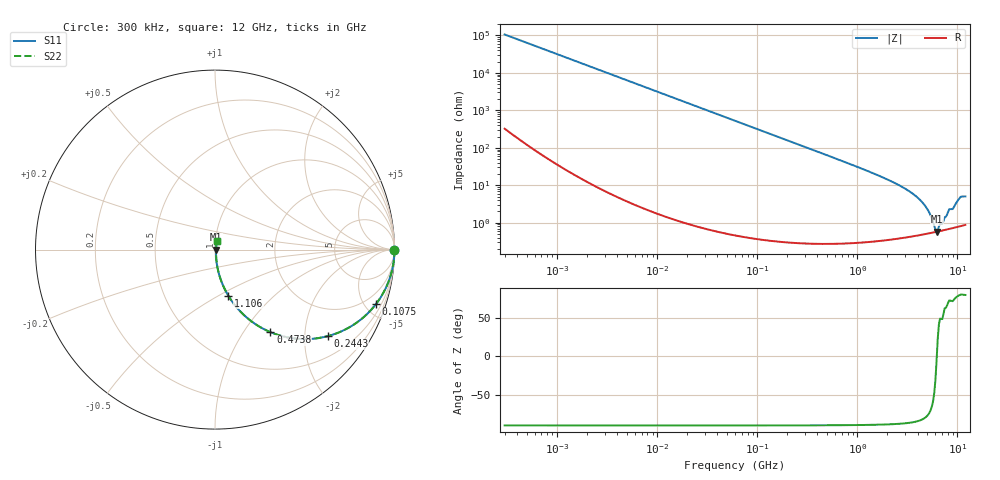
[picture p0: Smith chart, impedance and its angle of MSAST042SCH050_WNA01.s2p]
! MSAST042SCH050_WNA01  S-PARAMETER MODEL  ( General Type )
! Model Generated by TAIYO YUDEN Corporation (http://www.ty-top.com)
! Version 1.0
! TAIYO YUDEN Control No. 150820
! Copyright(c) 2015 TAIYO YUDEN CO.,LTD. All Rights Reserved.
! Product Description (link to TY-COMPAS)
! https://ds.yuden.co.jp/TYCOMPAS/or/detail?pn=MSAST042SCH050BWNA01&u=M
! Products Name : Multilayer Ceramic Capacitors
! Characteristics :
!  Capacitance : 5 pF , Rated Voltage : 25V , TCC : CH / C0H
!  Case Size : 0.4 x 0.2 / 0.016 x 0.008 [mm/inch] , Thickness : 0.2 / 0.008 [mm/inch]
!  (Conditions: Temperature = 25 degC , DC Bias Current/Voltage = 0A / 0V)
! External Node Assignments :
!  1  o---| |---o  2
! GND o---------o GND
! Frequency Range : 0.3MHz  -  12000MHz  [ 401 STEP ]
# MHz S RI R 50
! Freq[MHz].  S11 Real  S11 Imag  S21 Real  S21 Imag  S12 Real  S12 Imag  S22 Real  S22 Imag
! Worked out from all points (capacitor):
!   401 points, 300 kHz to 12 GHz, reference 50 ohm
!   read as one part in series: C = 5.01 pF near 316.3 kHz
!   lowest |Z| = 576 mohm at 6.188 GHz (marker M1)
!   series resonance near 6.217 GHz, so ESL is about 130 pH
!   S11 on the Smith chart (normalised r, x): 300 kHz: open; 107.5 MHz: 1.01, -5.91; 244.3 MHz: 1.01, -2.60; 473.8 MHz: 1.01, -1.33; 1.106 GHz: 1.01, -0.56; 12 GHz: 1.02, +0.10
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0.3  1 -0.000945  3.78e-06 0.000945  3.78e-06 0.000945  1 -0.000945
1.769972  1 -0.00557  3.56e-05 0.00557  3.56e-05 0.00557  1 -0.00557
10.44266  0.9989 -0.0328  0.0011 0.0328  0.0011 0.0328  0.9989 -0.0328
60  0.9654 -0.1824  0.0346 0.1824  0.0346 0.1824  0.9654 -0.1824
107.4644  0.8969 -0.3035  0.1031 0.3035  0.1031 0.3035  0.8969 -0.3035
244.3004  0.6272 -0.4824  0.3728 0.4824  0.3728 0.4824  0.6272 -0.4824
353.9943  0.4445 -0.4954  0.5555 0.4954  0.5555 0.4954  0.4445 -0.4954
473.7541  0.3083 -0.4597  0.6917 0.4597  0.6917 0.4597  0.3083 -0.4597
704.9044  0.1667 -0.3696  0.8333 0.3696  0.8333 0.3696  0.1667 -0.3696
1105.905  0.0741 -0.2567  0.9259 0.2567  0.9259 0.2567  0.0741 -0.2567
2088.533  0.0212 -0.1316  0.9788 0.1316  0.9788 0.1316  0.0212 -0.1316
3190.978  0.00939 -0.0724  0.9906 0.0724  0.9906 0.0724  0.00939 -0.0724
4270.516  0.00621 -0.0389  0.9938 0.0389  0.9938 0.0389  0.00621 -0.0389
5006.236  0.00557 -0.0222  0.9944 0.0222  0.9944 0.0222  0.00557 -0.0222
5420.343  0.00549 -0.014  0.9945 0.014  0.9945 0.014  0.00549 -0.014
5868.704  0.00557 -0.00595  0.9944 0.00595  0.9944 0.00595  0.00557 -0.00595
6188.031  0.0057 -0.000506  0.9943 0.000506  0.9943 0.000506  0.0057 -0.000506
6524.734  0.0059 0.00519  0.9941 -0.00519  0.9941 -0.00519  0.0059 0.00519
8064.993  0.00701 0.0182  0.993 -0.0182  0.993 -0.0182  0.00701 0.0182
9207.246  0.00788 0.0248  0.9921 -0.0248  0.9921 -0.0248  0.00788 0.0248
10511.28  0.00988 0.0441  0.9901 -0.0441  0.9901 -0.0441  0.00988 0.0441
12000  0.0111 0.0485  0.9889 -0.0485  0.9889 -0.0485  0.0111 0.0485
